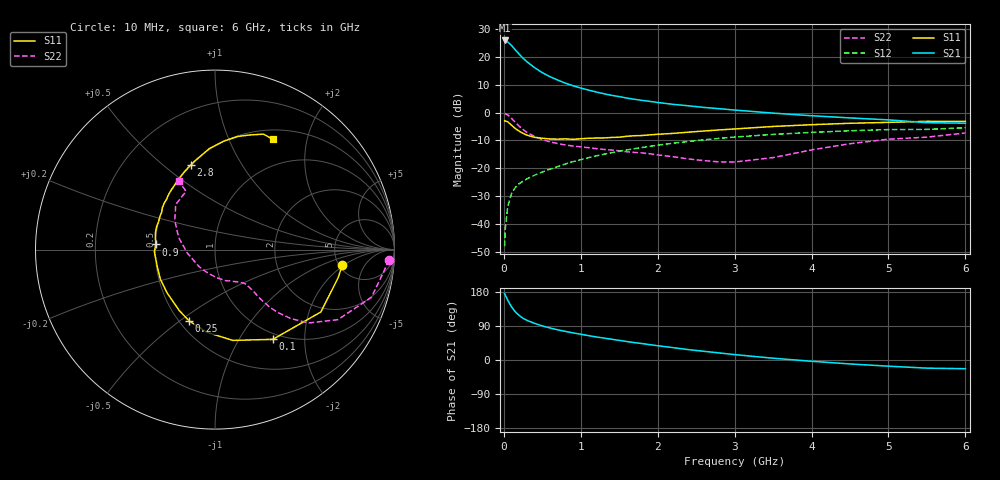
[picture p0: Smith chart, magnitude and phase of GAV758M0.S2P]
! Infineon Technologies  Discrete & RF Semiconductors
! BF775
! Si NPN RF Bipolar Junction Transistor in SOT23
! VCE = 0.75 V  IC = 8 mA
! Common Emitter S-Parameters:  May  1996
# GHz  S  MA  R  50
!  f  S11  S21  S12  S22
! GHz  MAG  ANG  MAG  ANG  MAG  ANG  MAG  ANG
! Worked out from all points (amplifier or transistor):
!   36 points, 10 MHz to 6 GHz, reference 50 ohm
!   highest |S21| = 25.9 dB at 10 MHz (marker M1)
!   |S21| within 3 dB of that: start of sweep to 136.9 MHz
!   unconditionally stable (mu >= 1): 508 MHz to end of sweep
!   at 250 MHz: K = 0.68, MSG = 22.1 dB, |S12| = -24.6 dB
!   at 1.4 GHz: K = 1.19, MAG = 7.7 dB, |S12| = -14.4 dB
!   at 6 GHz: K = 1.05, MAG = -0.6 dB, |S12| = -5.4 dB
!   S11 on the Smith chart (normalised r, x): 10 MHz: 5.37, -1.83; 100 MHz: 0.91, -1.41; 250 MHz: 0.56, -0.54; 900 MHz: 0.50, +0.03; 2.8 GHz: 0.50, +0.62; 6 GHz: 0.62, +1.46
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0.01  0.7149 -6.7  19.74 175.5  0.004 85.8  0.9685 -3.4
0.02  0.7041 -12.7  19.55 170.8  0.0085 84.6  0.9507 -7.0
0.05  0.6846 -30.5  18.63 158.1  0.0204 75.2  0.9109 -17.0
0.1  0.5949 -57.2  16.02 140.3  0.0355 64.6  0.7878 -29.7
0.15  0.5155 -78.9  13.31 126.7  0.0455 58.5  0.6637 -38.0
0.2  0.4634 -95.4  11.18 117.5  0.053 55.8  0.5705 -42.3
0.25  0.4231 -109.8  9.467 110.0  0.0589 54.3  0.4961 -45.0
0.3  0.3934 -120.5  8.182 104.6  0.0644 54.3  0.4419 -46.5
0.4  0.3597 -138.0  6.411 96.7  0.0753 54.8  0.3721 -47.4
0.5  0.3464 -151.4  5.208 90.0  0.0856 55.8  0.3276 -47.4
0.6  0.3362 -162.1  4.417 84.5  0.0967 56.8  0.2982 -47.5
0.7  0.3341 -171.0  3.84 79.6  0.1078 57.3  0.2779 -47.8
0.9  0.3312 175.0  3.033 71.6  0.1317 57.5  0.2511 -48.8
1.1  0.3457 163.3  2.539 64.4  0.1554 56.8  0.2346 -51.7
1.3  0.3509 153.5  2.182 57.9  0.1788 55.5  0.2183 -55.0
1.6  0.3759 141.2  1.821 48.7  0.2139 52.7  0.1982 -62.1
2.2  0.4231 122.2  1.407 32.6  0.2824 45.9  0.1615 -83.1
2.8  0.4887 106.2  1.175 18.6  0.3449 37.8  0.1304 -119.5
3.5  0.5637 93.2  0.979 4.7  0.4058 27.7  0.1558 -173.1
4.5  0.6433 78.5  0.803 -10.4  0.4723 14.0  0.2764 144.2
5.5  0.6978 67.2  0.659 -21.5  0.4991 0.6  0.3628 116.4
6  0.6939 62.5  0.646 -23.0  0.5347 -3.2  0.4301 117.7
